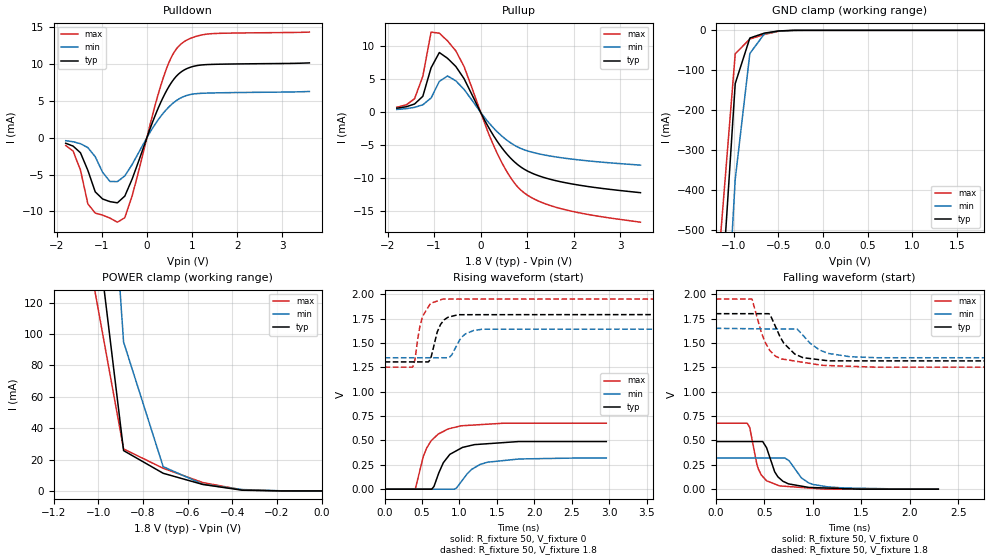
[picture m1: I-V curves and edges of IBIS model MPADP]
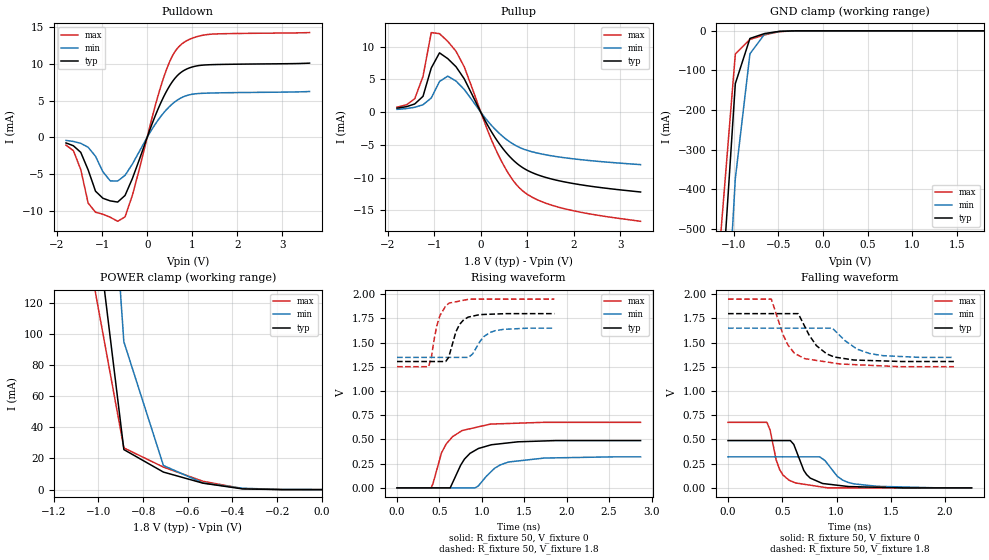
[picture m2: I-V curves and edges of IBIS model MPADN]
| Created by SiliconSmart 2008.10 (Production)
| There are several IBIS sections which it is inappropriate for this tool to
| automatically fill in - copyrights and packaging details are two examples.
| We are making it easy for you to add these things by providing commented-out
| section headers and brief descriptions of each such section.  Of course, the
| IBIS standard is the ultimate section description; these are merely summaries.
[IBIS Ver]   4.1
[File Name]   ar_all.ibs
[File Rev]   1.0
[Date]   December 18 11:22:04
[Source]   From SiliconSmart 2008.10 (Production)
|[Notes]   Use this section for any special notes related to the file.
|   (fill in and uncomment to use this section)
|[Disclaimer]   Legal disclaimer section.
|   (fill in and uncomment to use this section)
|[Copyright]   Copyright 1995, XYZ Corp., All Rights Reserved
|   (fill in and uncomment to use this section)
[Component]   pdqs_ddr2_cl_driver_6p9ma
[Manufacturer]   Unknown
[Package]
| Variable   typ   min   max
R_pkg   18   18   18
L_pkg   1n   1n   1n
C_pkg   15f   15f   15f
[Pin]   signal_name   model_name   R_pin   L_pin   C_pin
1   PADP   MPADP   NA   NA   NA
2   PADN   MPADN   NA   NA   NA
3   DVSS   GND   NA   NA   NA
4   DVDD   POWER   NA   NA   NA
|[Package Model]   Package model name.  40-char limit.
|   (fill in and uncomment to use this section)
[Pin Mapping]  pulldown_ref   pullup_ref   gnd_clamp_ref  power_clamp_ref
1   DVSS   DVDD   DVSS   DVDD
2   DVSS   DVDD   DVSS   DVDD
3   DVSS   NC   NC   NC
4   NC   DVDD   NC   NC
[Diff Pin]  inv_pin  vdiff  tdelay_typ tdelay_min tdelay_max
1   2   NA   -59.67p   -36.38p   -48.59p
| Models and submodels in the file (2): MPADP (I/O), MPADN (I/O)
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|PADP pin
[Model]   MPADP
Model_type I/O
Polarity Non-Inverting
Vinl = 0.8
Vinh = 2.0
Vmeas = 0.9
| Capacitance   typ   min   max
C_comp   6.42p   1.25p   1.25p
| Variables   typ   min   max
[Temperature Range]   25   125   -40
[Voltage Range]   1.8   1.65   1.95
[Pullup Reference]   1.8   1.65   1.95
[Pulldown Reference]   0.0   0.0   0.0
[POWER Clamp Reference]   1.8   1.65   1.95
[GND Clamp Reference]   0.0   0.0   0.0
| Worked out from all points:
|   slope of the pulldown table from 0 to 0.27 V, typ, clamps not added: 63.1 ohm
|   slope of the pullup table from 0 to 0.27 V, typ, clamps not added: 78.4 ohm
|   GND clamp passes 1 mA (typ) near -0.44 V on its own axis
|   POWER clamp passes 1 mA (typ) near -0.38 V on its own axis
|   falling waveform, R_fixture 50, V_fixture 0: 20-80 % time 138ps typ, 178ps min, 110ps max; typ from 0.489 V to 0 V
|   falling waveform, R_fixture 50, V_fixture 1.8: 20-80 % time 195ps typ, 230ps min, 175ps max; typ from 1.8 V to 1.3 V
|   rising waveform, R_fixture 50, V_fixture 0: 20-80 % time 260ps typ, 277ps min, 231ps max; typ from 0 V to 0.489 V
|   rising waveform, R_fixture 50, V_fixture 1.8: 20-80 % time 122ps typ, 156ps min, 120ps max; typ from 1.3 V to 1.8 V
[Pulldown]
| Voltage   I(typ)   I(min)   I(max)
-1.8V     -761.5uA   -413.9uA   -1.059mA
-1.636V   -1.146mA   -559.1uA   -1.817mA
-1.473V   -2.052mA   -817.8uA   -4.395mA
-1.309V   -4.439mA   -1.35mA    -8.977mA
-1.145V   -7.351mA   -2.589mA   -10.22mA
-818.2mV  -8.675mA   -5.944mA   -10.91mA
-654.5mV  -8.833mA   -5.963mA   -11.46mA
-490.9mV  -7.931mA   -5.192mA   -10.86mA
337.5mV   5.186mA    3.132mA    7.644mA
731.2mV   8.779mA    5.321mA    12.56mA
1.378V    9.913mA    6.045mA    14.06mA
3.6V      10.13mA    6.258mA    14.31mA
[GND Clamp]
| Voltage   I(typ)   I(min)   I(max)
-1.8V     -4.426A    -4.674A    -4.304A
-1.145V   -702.1mA   -1.023A    -514.4mA
-981.8mV  -133.3mA   -373.2mA   -58.54mA
-818.2mV  -19.27mA   -58.01mA   -21.8mA
-654.5mV  -6.911mA   -8.539mA   -10.26mA
-490.9mV  -1.444mA   -1.513mA   -2.127mA
-327.3mV  -103.9uA   -141.6uA   -116.5uA
1.8V      26.57nA    10.37uA    9.43nA
[Pullup]
| Voltage   I(typ)   I(min)   I(max)
-1.8V     617.4uA    424.5uA    761.5uA
-1.418V   1.248mA    741.4uA    2.053mA
-1.241V   2.414mA    1.129mA    5.452mA
-1.064V   6.729mA    2.155mA    12.14mA
-886.4mV  9.041mA    4.674mA    11.97mA
-709.1mV  8.162mA    5.492mA    10.8mA
-354.5mV  5.083mA    3.458mA    6.913mA
309.4mV   -3.883mA   -2.612mA   -5.489mA
590.6mV   -6.529mA   -4.36mA    -9.29mA
843.8mV   -8.182mA   -5.414mA   -11.64mA
1.688V    -10.47mA   -6.838mA   -14.52mA
3.436V    -12.18mA   -8.006mA   -16.65mA
[POWER Clamp]
| Voltage   I(typ)   I(min)   I(max)
-1.8V     4.331A     4.441A     4.305A
-1.773V   4.155A     4.271A     4.127A
-1.595V   3.037A     3.189A     2.978A
-1.418V   1.962A     2.154A     1.871A
-1.241V   976.7mA    1.208A     867.8mA
-1.064V   234.9mA    462.7mA    165.8mA
-886.4mV  25.71mA    94.99mA    26.78mA
-709.1mV  11.25mA    15.47mA    14.45mA
-531.8mV  4.13mA     4.272mA    5.343mA
-354.5mV  447.2uA    869.6uA    634.7uA
-177.3mV  4.06uA     65.5uA     3.418uA
0V        0A         0A         14.04nA
[Ramp]
dV/dt_r   0.29804/0.194218n 0.192315/0.276927n 0.41881/0.120325n
dV/dt_f   0.298045/0.170971n 0.181166/0.23008n 0.406106/0.11048n
R_load = 50
[Falling Waveform]
R_fixture = 50
V_fixture = 0
V_fixture_min = 0
V_fixture_max = 0
| Time   V(typ)   V(min)   V(max)
0s        488.5mV    320.6mV    676.9mV
324.2ps   488.5mV    320.6mV    676.9mV
350.7ps   488.5mV    320.6mV    632mV
423.7ps   488.5mV    320.6mV    256.5mV
469.4ps   488.5mV    320.6mV    145.6mV
657.3ps   112.1mV    320.6mV    33.64mV
757.3ps   53mV       290.7mV    26.48mV
883.7ps   31.09mV    114.8mV    17.43mV
1.004ns   16.42mV    48.22mV    8.801mV
2.295ns   24.89uV    44.78uV    21.07uV
[Falling Waveform]
R_fixture = 50
V_fixture = 1.8
V_fixture_min = 1.65
V_fixture_max = 1.95
| Time   V(typ)   V(min)   V(max)
0s        1.8V       1.65V      1.95V
374.1ps   1.8V       1.646V     1.95V
504.9ps   1.8V       1.644V     1.515V
561.7ps   1.788V     1.643V     1.418V
678.1ps   1.537V     1.643V     1.336V
840.7ps   1.374V     1.642V     1.31V
899.4ps   1.349V     1.578V     1.301V
1.157ns   1.317V     1.393V     1.268V
1.631ns   1.316V     1.349V     1.252V
31.56ns   1.305V     1.348V     1.252V
[Rising Waveform]
R_fixture = 50
V_fixture = 0
V_fixture_min = 0
V_fixture_max = 0
| Time   V(typ)   V(min)   V(max)
0s        24.6uV     45.5uV     21.3uV
409.1ps   24.6uV     45.5uV     21.3uV
560.4ps   24.6uV     45.5uV     420.1mV
659.3ps   27.87mV    45.5uV     524.1mV
783.7ps   270.9mV    45.5uV     592mV
849.3ps   335.5mV    45.5uV     617.8mV
960.6ps   394.7mV    12.32mV    638.8mV
1.162ns   450.1mV    202.5mV    656.6mV
1.377ns   466.3mV    276.8mV    666.6mV
2.962ns   488.5mV    320.6mV    676.9mV
[Rising Waveform]
R_fixture = 50
V_fixture = 1.8
V_fixture_min = 1.65
V_fixture_max = 1.95
| Time   V(typ)   V(min)   V(max)
0s        1.305V     1.348V     1.252V
373.6ps   1.305V     1.348V     1.252V
506.1ps   1.305V     1.348V     1.772V
606ps     1.327V     1.348V     1.897V
702.4ps   1.611V     1.348V     1.93V
776.8ps   1.719V     1.348V     1.95V
869.7ps   1.768V     1.355V     1.95V
1.078ns   1.79V      1.592V     1.95V
1.305ns   1.79V      1.641V     1.95V
31.56ns   1.8V       1.65V      1.95V
|PADN pin
[Model]   MPADN
Model_type I/O
Polarity Inverting
Vinl = 0.8
Vinh = 2.0
Vmeas = 0.9
| Capacitance   typ   min   max
C_comp   6.42p   1.25p   1.25p
| Variables   typ   min   max
[Temperature Range]   25   125   -40
[Voltage Range]   1.8   1.65   1.95
[Pullup Reference]   1.8   1.65   1.95
[Pulldown Reference]   0.0   0.0   0.0
[POWER Clamp Reference]   1.8   1.65   1.95
[GND Clamp Reference]   0.0   0.0   0.0
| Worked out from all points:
|   slope of the pulldown table from 0 to 0.27 V, typ, clamps not added: 63.1 ohm
|   slope of the pullup table from 0 to 0.27 V, typ, clamps not added: 78.4 ohm
|   GND clamp passes 1 mA (typ) near -0.44 V on its own axis
|   POWER clamp passes 1 mA (typ) near -0.38 V on its own axis
|   falling waveform, R_fixture 50, V_fixture 0: 20-80 % time 138ps typ, 178ps min, 107ps max; typ from 0.489 V to 0 V
|   falling waveform, R_fixture 50, V_fixture 1.8: 20-80 % time 195ps typ, 237ps min, 171ps max; typ from 1.8 V to 1.3 V
|   rising waveform, R_fixture 50, V_fixture 0: 20-80 % time 249ps typ, 279ps min, 224ps max; typ from 0 V to 0.489 V
|   rising waveform, R_fixture 50, V_fixture 1.8: 20-80 % time 123ps typ, 161ps min, 114ps max; typ from 1.3 V to 1.8 V
[Pulldown]
| Voltage   I(typ)   I(min)   I(max)
-1.8V     -761.5uA   -413.9uA   -1.059mA
-1.636V   -1.146mA   -559.1uA   -1.817mA
-1.473V   -2.052mA   -817.8uA   -4.395mA
-1.309V   -4.439mA   -1.35mA    -8.977mA
-1.145V   -7.351mA   -2.589mA   -10.22mA
-818.2mV  -8.675mA   -5.944mA   -10.91mA
-654.5mV  -8.833mA   -5.963mA   -11.46mA
-490.9mV  -7.931mA   -5.192mA   -10.86mA
337.5mV   5.186mA    3.132mA    7.644mA
731.2mV   8.779mA    5.321mA    12.56mA
1.378V    9.913mA    6.045mA    14.06mA
3.6V      10.13mA    6.258mA    14.31mA
[GND Clamp]
| Voltage   I(typ)   I(min)   I(max)
-1.8V     -4.426A    -4.674A    -4.304A
-1.145V   -702.1mA   -1.023A    -514.4mA
-981.8mV  -133.3mA   -373.2mA   -58.54mA
-818.2mV  -19.27mA   -58.01mA   -21.8mA
-654.5mV  -6.911mA   -8.539mA   -10.26mA
-490.9mV  -1.444mA   -1.513mA   -2.127mA
-327.3mV  -103.9uA   -141.6uA   -116.5uA
1.8V      26.57nA    10.37uA    9.43nA
[Pullup]
| Voltage   I(typ)   I(min)   I(max)
-1.8V     617.4uA    424.5uA    761.5uA
-1.418V   1.248mA    741.4uA    2.053mA
-1.241V   2.414mA    1.129mA    5.452mA
-1.064V   6.729mA    2.155mA    12.14mA
-886.4mV  9.041mA    4.674mA    11.97mA
-709.1mV  8.162mA    5.492mA    10.8mA
-354.5mV  5.083mA    3.458mA    6.913mA
309.4mV   -3.883mA   -2.612mA   -5.489mA
590.6mV   -6.529mA   -4.36mA    -9.29mA
843.8mV   -8.182mA   -5.414mA   -11.64mA
1.688V    -10.47mA   -6.838mA   -14.52mA
3.436V    -12.18mA   -8.006mA   -16.65mA
[POWER Clamp]
| Voltage   I(typ)   I(min)   I(max)
-1.8V     4.331A     4.441A     4.305A
-1.773V   4.155A     4.271A     4.127A
-1.595V   3.037A     3.189A     2.978A
-1.418V   1.962A     2.154A     1.871A
-1.241V   976.7mA    1.208A     867.8mA
-1.064V   234.9mA    462.7mA    165.8mA
-886.4mV  25.71mA    94.99mA    26.78mA
-709.1mV  11.25mA    15.47mA    14.45mA
-531.8mV  4.13mA     4.272mA    5.343mA
-354.5mV  447.2uA    869.6uA    634.7uA
-177.3mV  4.06uA     65.5uA     3.418uA
0V        0A         0A         14.04nA
[Ramp]
dV/dt_r   0.29804/0.191752n 0.192315/0.279035n 0.41881/0.11394n
dV/dt_f   0.298045/0.170954n 0.181166/0.236573n 0.406106/0.106907n
R_load = 50
[Falling Waveform]
R_fixture = 50
V_fixture = 0
V_fixture_min = 0
V_fixture_max = 0
| Time   V(typ)   V(min)   V(max)
0s        488.5mV    320.6mV    676.9mV
358.7ps   488.5mV    320.6mV    676.9mV
476.3ps   488.5mV    320.6mV    186.9mV
574.4ps   488.5mV    320.6mV    73.56mV
622.5ps   400.9mV    320.6mV    50.65mV
724.8ps   136.5mV    320.6mV    33.15mV
871.5ps   44.96mV    299.2mV    8.046mV
1.006ns   27.3mV     120.7mV    21.19uV
1.162ns   12.01mV    40.87mV    21.19uV
2.244ns   25.08uV    45.5uV     21.19uV
[Falling Waveform]
R_fixture = 50
V_fixture = 1.8
V_fixture_min = 1.65
V_fixture_max = 1.95
| Time   V(typ)   V(min)   V(max)
0s        1.8V       1.65V      1.95V
399ps     1.8V       1.65V      1.95V
552.9ps   1.8V       1.65V      1.475V
647.3ps   1.8V       1.65V      1.37V
707.3ps   1.667V     1.65V      1.335V
814.1ps   1.47V      1.65V      1.317V
981.2ps   1.351V     1.628V     1.289V
1.189ns   1.32V      1.434V     1.272V
1.305ns   1.316V     1.388V     1.266V
2.082ns   1.305V     1.348V     1.252V
[Rising Waveform]
R_fixture = 50
V_fixture = 0
V_fixture_min = 0
V_fixture_max = 0
| Time   V(typ)   V(min)   V(max)
0s        24.59uV    45.51uV    20.89uV
402.7ps   24.59uV    45.51uV    20.89uV
524.1ps   24.59uV    45.51uV    360.8mV
579.2ps   24.59uV    45.51uV    453mV
627.1ps   24.59uV    45.51uV    500.8mV
769.2ps   260.8mV    45.51uV    592.6mV
959.6ps   406.9mV    20.69mV    630.5mV
1.15ns    449mV      202.1mV    660.2mV
1.315ns   465mV      267.3mV    665.1mV
2.871ns   488.5mV    320.6mV    676.9mV
[Rising Waveform]
R_fixture = 50
V_fixture = 1.8
V_fixture_min = 1.65
V_fixture_max = 1.95
| Time   V(typ)   V(min)   V(max)
0s        1.305V     1.348V     1.252V
372.3ps   1.305V     1.348V     1.252V
405.8ps   1.305V     1.348V     1.35V
468.6ps   1.305V     1.348V     1.673V
505ps     1.305V     1.348V     1.778V
615.8ps   1.369V     1.348V     1.909V
735.5ps   1.686V     1.348V     1.93V
838.5ps   1.764V     1.348V     1.948V
1.099ns   1.794V     1.606V     1.95V
1.856ns   1.8V       1.65V      1.95V
